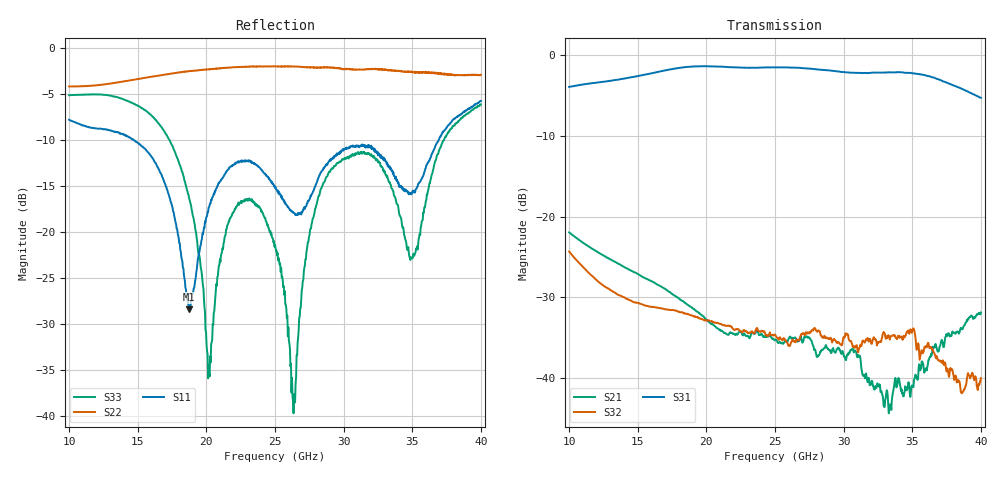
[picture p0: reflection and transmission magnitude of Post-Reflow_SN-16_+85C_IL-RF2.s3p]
!Agilent Technologies,N5245A,US49150155,A.09.90.19
!Agilent N5245A: A.09.90.19
!Date: Wednesday, November 14, 2018 03:51:09
!Correction: S11(Full 3 Port(1,2,3))
!S12(Full 3 Port(1,2,3))
!S13(Full 3 Port(1,2,3))
!S21(Full 3 Port(1,2,3))
!S22(Full 3 Port(1,2,3))
!S23(Full 3 Port(1,2,3))
!S31(Full 3 Port(1,2,3))
!S32(Full 3 Port(1,2,3))
!S33(Full 3 Port(1,2,3))
!S3P File: Measurements: <S11,S12,S13>,
!<S21,S22,S23>,
!<S31,S32,S33>:
# Hz S  dB  R 50
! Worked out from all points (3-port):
!   801 points, 10 GHz to 40 GHz, reference 50 ohm
!   strongest paths, dB at 10 GHz, 17.5 GHz, 25 GHz, 32.5 GHz, 40 GHz:
!     S31: -3.9, -1.7, -1.5, -2.1, -5.3
!     S32: -24.3, -31.6, -34.6, -35.5, -40.0
!     S21: -22.0, -29.6, -35.3, -41.0, -31.9
!   lowest |S11| = -28.4 dB at 18.74 GHz (marker M1), VSWR 1.08, Z = 46.6 - j1.37 ohm
!   |S11| at or under -10 dB: 14.69 GHz to 36.93 GHz (22.24 GHz wide, 86.2 % of centre)
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1e10  -7.82 8.3  -21.96 91.4  -3.93 -160.0
      -21.95 91.4  -4.20 60.6  -24.34 23.4
      -3.93 -159.9  -24.33 23.5  -5.15 -104.2
1.50625e10  -10.42 -142.3  -27.14 -3.8  -2.57 91.9
            -27.16 -3.6  -3.38 -40.1  -30.73 -70.0
            -2.56 92.0  -30.71 -69.9  -6.34 165.0
1.87375e10  -28.38 -157.3  -31.04 -71.3  -1.44 9.5
            -31.05 -71.1  -2.54 -98.1  -32.15 -147.2
            -1.44 9.7  -32.12 -147.0  -16.29 95.4
2.01625e10  -17.34 -110.2  -32.99 -92.9  -1.37 -23.6
            -33.01 -93.0  -2.35 -117.4  -32.88 -178.4
            -1.36 -23.4  -32.87 -178.2  -34.50 136.3
2.21875e10  -12.50 -141.7  -34.51 -112.2  -1.52 -69.1
            -34.51 -112.7  -2.11 -142.1  -33.93 136.5
            -1.51 -69.0  -33.91 136.7  -17.31 -174.6
2.5e10  -15.22 -176.6  -35.36 -154.6  -1.51 -131.4
        -35.34 -155.0  -2.01 -174.2  -34.64 71.2
        -1.50 -131.2  -34.61 71.4  -21.37 118.4
2.635e10  -17.91 -170.4  -35.08 -173.0  -1.54 -162.2
          -35.08 -173.4  -2.03 170.5  -35.41 45.7
          -1.54 -162.0  -35.42 46.2  -39.67 12.6
3.0925e10  -10.60 179.0  -36.81 99.1  -2.21 94.0
           -36.83 99.9  -2.39 114.4  -36.01 -61.1
           -2.20 94.3  -35.95 -60.4  -11.49 170.9
3.49375e10  -15.91 161.8  -41.12 87.6  -2.23 -3.0
            -41.11 87.3  -2.67 55.7  -34.32 -163.2
            -2.22 -2.7  -34.26 -163.2  -22.75 2.0
4e10  -5.77 121.5  -31.87 -4.8  -5.30 -132.9
      -31.88 -4.8  -2.94 -26.9  -40.25 -21.2
      -5.28 -132.5  -40.02 -21.7  -6.15 134.4
